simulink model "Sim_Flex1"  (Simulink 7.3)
settings: Solver=ode23  StartTime=0.0  StopTime=120  FixedStep=Ts  RelTol=1e-3
InitFcn:
  | r2d= 180/pi; d2r=1/r2d; Ts=0.04;                  % Radian to degree converts
  | [Afls,Bfls,Cfls,Dfls]= vehicle_flex_s;            % Shuttle Ascent, Max_Q, T=55 sec, Flex Vehicle with Slosh and TWD
  | [Aflz,Bflz,Cflz,Dflz]= vehicle_flex_z;            % Discrete Shuttle Plant Model at Max-Q (Flex Vehicle, Actuators, Sensors)
  | [Alfc,Blfc,Clfc,Dlfc]= lateral_fcs;               % Lateral Flight Control System
  | [Apfc,Bpfc,Cpfc,Dpfc]= pitch_fcs;                 % Pitch Flight Control System
  | [Azpl,Bzpl,Czpl,Dzpl]= vehi_plant_z;              % Load Discrete Plant (Vehi,Actuat,Sensors)
  | [Acts,Bcts,Ccts,Dcts]= actuators_5s;              % System of Five Actuators
  | [Actz,Bctz,Cctz,Dctz]= actuators_5z;              % System of Five Actuators, Z-Transform
  | [Asz, Bsz, Csz, Dsz] = sensors_z;                 % IMU, Gyro, Accelerometer Sensors, Z-transform
  | [Aol, Bol, Col, Dol] = open_loop;                 % Open-Loop System (Plant + FCS)
  | load TVC.Mat -ascii                               % Shuttle Stage-1 TVC Matrix at Max-Q
StopFcn:
  | Pl
undefined symbols (not defined in the file or in its folder): Acts, Afls, Alfc, Apfc, Asz, Bcts, Bfls, Blfc, Bpfc, Bsz, Ccts, Cfls, Clfc, Cpfc, Csz, Dcts, Dfls, Dlfc, Dpfc, Dsz, TVC

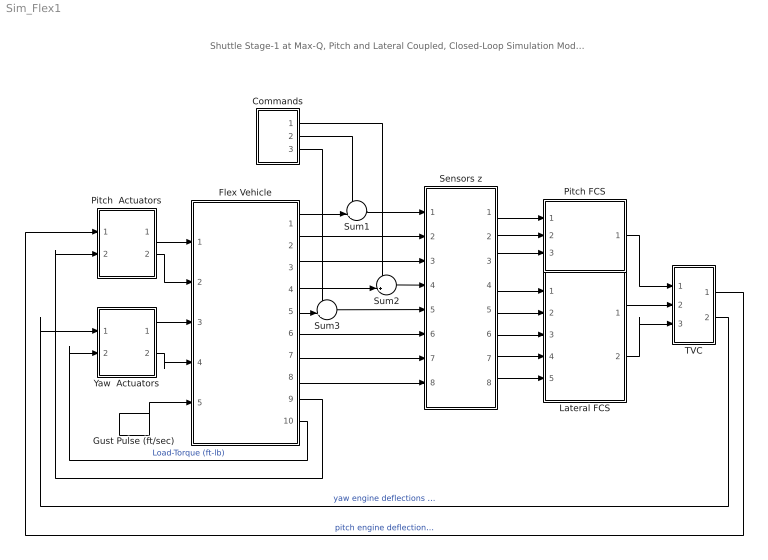
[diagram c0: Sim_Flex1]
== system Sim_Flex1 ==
  note: Shuttle Stage-1 at Max-Q, Pitch and Lateral Coupled, Closed-Loop Simulation Model-1
  Commands : Subsystem
  Flex Vehicle : Subsystem
  Gust Pulse (ft/sec) : DiscretePulseGenerator  PulseType=Time based  Amplitude=30  Period=200  PulseWidth=2.0  PhaseDelay=0.12  SampleTime=1
  Lateral FCS : Subsystem
  Pitch  Actuators : Subsystem
  Pitch FCS : Subsystem
  Sensors z : Subsystem
  Sum1 : Sum  Inputs=-+|  OutDataType=sfix(16)  OutScaling=2^0
  Sum2 : Sum  Inputs=-+|  OutDataType=sfix(16)  OutScaling=2^0
  Sum3 : Sum  Inputs=-+|  OutDataType=sfix(16)  OutScaling=2^0
  TVC : Subsystem
  Yaw  Actuators : Subsystem
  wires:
  Gust Pulse (ft/sec)/1 -> Flex Vehicle/5(WG)
  Flex Vehicle/2(q-flx) -> Sensors z/2(qi)
  Flex Vehicle/3(Nz) -> Sensors z/3(Nzi)
  Flex Vehicle/6(p-flx) -> Sensors z/6(pi)
  Flex Vehicle/7(r-flx) -> Sensors z/7(ri)
  Flex Vehicle/8(Ny) -> Sensors z/8(Nyi)
  Sensors z/1(theo) -> Pitch FCS/1(theta)
  Sensors z/2(qo) -> Pitch FCS/2(q)
  Sensors z/3(Nzo) -> Pitch FCS/3(Nz)
  Sensors z/4(pho) -> Lateral FCS/1(phi-er)
  Sensors z/5(pso) -> Lateral FCS/2(psi-er)
  Sensors z/6(po) -> Lateral FCS/3(p)
  Sensors z/7(ro) -> Lateral FCS/4(r)
  Sensors z/8(Nyo) -> Lateral FCS/5(Ny)
  Pitch  Actuators/1(dy) -> Flex Vehicle/1(dy)
  Yaw  Actuators/1(dz) -> Flex Vehicle/3(dz)
  Yaw  Actuators/2(dzdd) -> Flex Vehicle/4(dzdd)
  Pitch  Actuators/2(dydd) -> Flex Vehicle/2(dydd)
  Flex Vehicle/1(theta) -> Sum1/2
  Sum1/1 -> Sensors z/1(thei)
  Flex Vehicle/4(phi) -> Sum2/2
  Sum2/1 -> Sensors z/4(phi)
  Flex Vehicle/10(TLz) -> Yaw  Actuators/2(TLz)  "Load-Torque (ft-lb)"
  Flex Vehicle/9(TLy) -> Pitch  Actuators/2(TLy)
  Lateral FCS/1(DP_TVC) -> TVC/2(roll)
  Lateral FCS/2(DR_TVC) -> TVC/3(yaw)
  Pitch FCS/1(DQ_TVC) -> TVC/1(ptch)
  TVC/2(dz) -> Yaw  Actuators/1(dzc)  "yaw engine deflections (rad)"
  TVC/1(dy) -> Pitch  Actuators/1(dyc)  "pitch engine deflections (rad)"
  Sum3/1 -> Sensors z/5("psi ")
  Flex Vehicle/5(psi) -> Sum3/2
  Commands/1(roll) -> Sum2/1
  Commands/3(yaw) -> Sum3/1
  Commands/2(ptch) -> Sum1/1

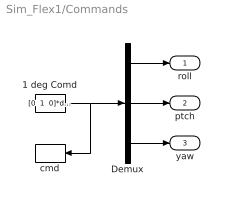
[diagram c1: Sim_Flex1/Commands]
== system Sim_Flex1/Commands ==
  1 deg Comd : Constant  Value="[0  1  0]*d2r"  OutDataType=sfix(16)  OutScaling=2^0  SampleTime=-1
  Demux : Demux  Outputs=3
  cmd : ToWorkspace  VariableName=cmd  SampleTime=-1  SaveFormat=Array
  roll : Outport
  ptch : Outport  Port=2
  yaw : Outport  Port=3
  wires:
  1 deg Comd/1 -> Demux/1, cmd/1
  Demux/1 -> roll/1
  Demux/2 -> ptch/1
  Demux/3 -> yaw/1

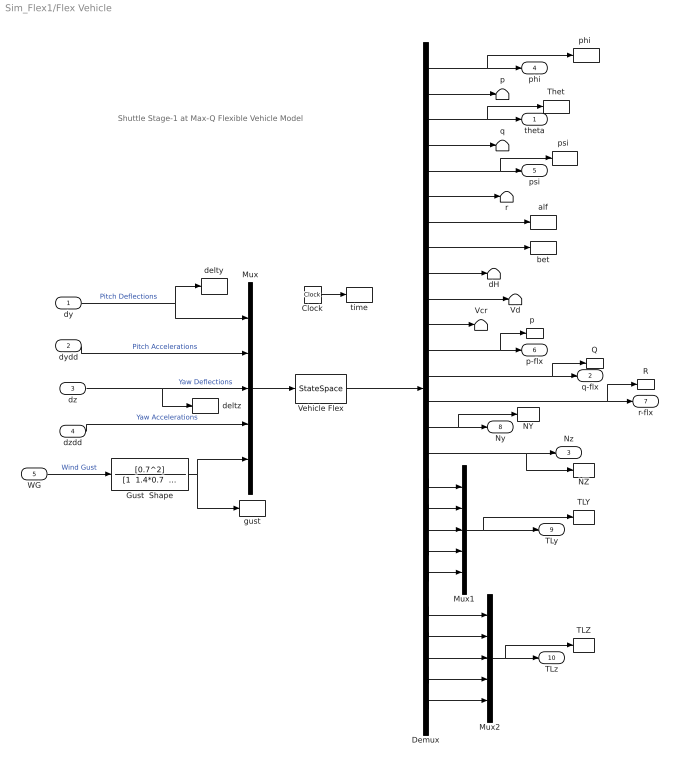
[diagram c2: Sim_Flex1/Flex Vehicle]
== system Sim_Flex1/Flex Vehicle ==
  note: Shuttle Stage-1 at Max-Q Flexible Vehicle Model
  dy : Inport  PortDimensions=5  OutDataType=sfix(16)  OutScaling=2^0
  dydd : Inport  Port=2  PortDimensions=5  OutDataType=sfix(16)  OutScaling=2^0
  dz : Inport  Port=3  PortDimensions=5  OutDataType=sfix(16)  OutScaling=2^0
  dzdd : Inport  Port=4  PortDimensions=5  OutDataType=sfix(16)  OutScaling=2^0
  WG : Inport  Port=5  OutDataType=sfix(16)  OutScaling=2^0
  Clock : Clock
  Demux : Demux  Outputs=26
  Gust  Shape : TransferFcn  Numerator=[0.7^2]  Denominator="[1  1.4*0.7  0.7^2]"
  Mux : Mux  Inputs="[5  5  5  5  1]"
  Mux1 : Mux  Inputs=5
  Mux2 : Mux  Inputs=5
  NY : ToWorkspace  VariableName=Ny  SampleTime=-1  SaveFormat=Array
  NZ : ToWorkspace  VariableName=Nz  SampleTime=-1  SaveFormat=Array
  Q : ToWorkspace  VariableName=q  SampleTime=-1  SaveFormat=Array
  R : ToWorkspace  VariableName=r  SampleTime=-1  SaveFormat=Array
  TLY : ToWorkspace  VariableName=TLy  SampleTime=-1  SaveFormat=Array
  TLZ : ToWorkspace  VariableName=TLz  SampleTime=-1  SaveFormat=Array
  Thet : ToWorkspace  VariableName=theta  SampleTime=-1  SaveFormat=Array
  Vcr : Terminator
  Vd : Terminator
  Vehicle Flex : StateSpace  A=Afls  B=Bfls  C=Cfls  D=Dfls
  alf : ToWorkspace  VariableName=alpha  SampleTime=-1  SaveFormat=Array
  bet : ToWorkspace  VariableName=beta  SampleTime=-1  SaveFormat=Array
  dH : Terminator
  delty : ToWorkspace  VariableName=delty  SampleTime=-1  SaveFormat=Array
  deltz : ToWorkspace  VariableName=deltz  SampleTime=-1  SaveFormat=Array
  gust : ToWorkspace  VariableName=Gust  SampleTime=-1  SaveFormat=Array
  p : Terminator
  "p  " : ToWorkspace  VariableName=p  SampleTime=-1  SaveFormat=Array
  "phi " : ToWorkspace  VariableName=phi  SampleTime=-1  SaveFormat=Array
  "psi " : ToWorkspace  VariableName=psi  SampleTime=-1  SaveFormat=Array
  q : Terminator
  r : Terminator
  time : ToWorkspace  VariableName=time  SampleTime=-1  SaveFormat=Array
  theta : Outport  OutDataType=sfix(16)  OutScaling=2^0
  q-flx : Outport  Port=2  OutDataType=sfix(16)  OutScaling=2^0
  Nz : Outport  Port=3  OutDataType=sfix(16)  OutScaling=2^0
  phi : Outport  Port=4  OutDataType=sfix(16)  OutScaling=2^0
  psi : Outport  Port=5  OutDataType=sfix(16)  OutScaling=2^0
  p-flx : Outport  Port=6  OutDataType=sfix(16)  OutScaling=2^0
  r-flx : Outport  Port=7  OutDataType=sfix(16)  OutScaling=2^0
  Ny : Outport  Port=8  OutDataType=sfix(16)  OutScaling=2^0
  TLy : Outport  Port=9  OutDataType=sfix(16)  OutScaling=2^0
  TLz : Outport  Port=10  OutDataType=sfix(16)  OutScaling=2^0
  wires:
  Mux/1 -> Vehicle Flex/1
  WG/1 -> Gust  Shape/1  "Wind Gust"
  dz/1 -> Mux/3, deltz/1  "Yaw Deflections"
  dydd/1 -> Mux/2  "Pitch Accelerations"
  dy/1 -> Mux/1, delty/1  "Pitch Deflections"
  Demux/1 -> phi/1, "phi "/1
  Demux/5 -> psi/1, "psi "/1
  Demux/2 -> p/1
  Demux/6 -> r/1
  Demux/8 -> bet/1
  Demux/12 -> p-flx/1, "p  "/1
  Demux/13 -> q-flx/1, Q/1
  Demux/15 -> Ny/1, NY/1
  Demux/3 -> theta/1, Thet/1
  Demux/4 -> q/1
  Demux/7 -> alf/1
  Demux/11 -> Vcr/1
  Demux/10 -> Vd/1
  Demux/9 -> dH/1
  Demux/14 -> r-flx/1, R/1
  Demux/16 -> Nz/1, NZ/1
  dzdd/1 -> Mux/4  "Yaw Accelerations"
  Demux/21 -> Mux1/5
  Demux/20 -> Mux1/4
  Demux/19 -> Mux1/3
  Demux/18 -> Mux1/2
  Demux/17 -> Mux1/1
  Demux/22 -> Mux2/1
  Demux/23 -> Mux2/2
  Demux/24 -> Mux2/3
  Demux/25 -> Mux2/4
  Demux/26 -> Mux2/5
  Clock/1 -> time/1
  Mux1/1 -> TLY/1, TLy/1
  Mux2/1 -> TLZ/1, TLz/1
  Gust  Shape/1 -> Mux/5, gust/1
  Vehicle Flex/1 -> Demux/1

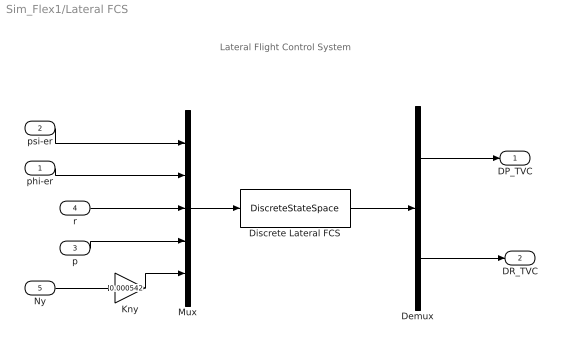
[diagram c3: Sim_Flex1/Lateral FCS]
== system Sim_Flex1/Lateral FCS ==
  note: Lateral Flight Control System
  phi-er : Inport  OutDataType=sfix(16)  OutScaling=2^0
  psi-er : Inport  Port=2  OutDataType=sfix(16)  OutScaling=2^0
  p : Inport  Port=3  OutDataType=sfix(16)  OutScaling=2^0
  r : Inport  Port=4  OutDataType=sfix(16)  OutScaling=2^0
  Ny : Inport  Port=5  OutDataType=sfix(16)  OutScaling=2^0
  Demux : Demux  Outputs=2
  Discrete Lateral FCS : DiscreteStateSpace  A=Alfc  B=Blfc  C=Clfc  D=Dlfc  SampleTime=Ts
  Kny : Gain  Gain=0.000542  ParameterDataType=sfix(16)  ParameterScaling=2^0  OutDataType=sfix(16)  OutScaling=2^0
  Mux : Mux  Inputs=5
  DP_TVC : Outport  OutDataType=sfix(16)  OutScaling=2^0
  DR_TVC : Outport  Port=2  OutDataType=sfix(16)  OutScaling=2^0
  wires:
  psi-er/1 -> Mux/1
  phi-er/1 -> Mux/2
  r/1 -> Mux/3
  Mux/1 -> Discrete Lateral FCS/1
  Discrete Lateral FCS/1 -> Demux/1
  Demux/1 -> DP_TVC/1
  Demux/2 -> DR_TVC/1
  p/1 -> Mux/4
  Ny/1 -> Kny/1
  Kny/1 -> Mux/5

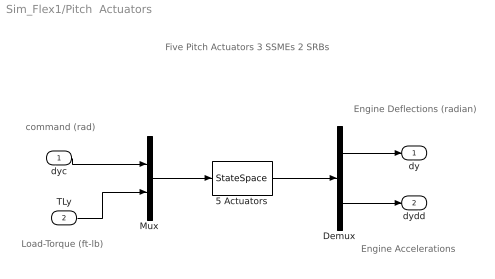
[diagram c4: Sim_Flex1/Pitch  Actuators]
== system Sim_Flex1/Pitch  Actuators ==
  note: Engine Accelerations
  note: Engine Deflections (radian)
  note: Five Pitch Actuators 3 SSMEs 2 SRBs
  note: Load-Torque (ft-lb)
  note: command (rad)
  dyc : Inport  OutDataType=sfix(16)  OutScaling=2^0
  TLy : Inport  Port=2  OutDataType=sfix(16)  OutScaling=2^0
  5 Actuators : StateSpace  A=Acts  B=Bcts  C=Ccts  D=Dcts
  Demux : Demux  Outputs=[5, 5]
  Mux : Mux  Inputs="[5  5]"
  dy : Outport  OutDataType=sfix(16)  OutScaling=2^0
  dydd : Outport  Port=2  OutDataType=sfix(16)  OutScaling=2^0
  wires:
  Mux/1 -> 5 Actuators/1
  dyc/1 -> Mux/1
  TLy/1 -> Mux/2
  Demux/1 -> dy/1
  Demux/2 -> dydd/1
  5 Actuators/1 -> Demux/1

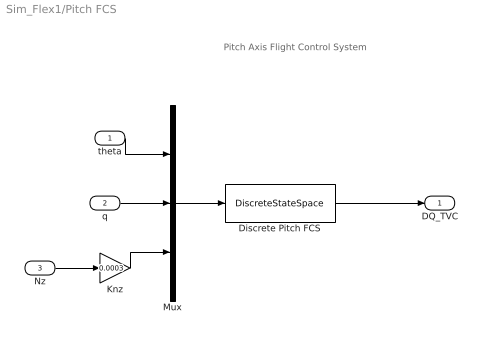
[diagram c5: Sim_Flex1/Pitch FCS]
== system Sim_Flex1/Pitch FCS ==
  note: Pitch Axis Flight Control System
  theta : Inport  OutDataType=sfix(16)  OutScaling=2^0
  q : Inport  Port=2  OutDataType=sfix(16)  OutScaling=2^0
  Nz : Inport  Port=3  OutDataType=sfix(16)  OutScaling=2^0
  Discrete Pitch FCS : DiscreteStateSpace  A=Apfc  B=Bpfc  C=Cpfc  D=Dpfc  SampleTime=Ts
  Knz : Gain  Gain=0.0003  ParameterDataType=sfix(16)  ParameterScaling=2^0  OutDataType=sfix(16)  OutScaling=2^0
  Mux : Mux  Inputs=3
  DQ_TVC : Outport  OutDataType=sfix(16)  OutScaling=2^0
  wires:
  Mux/1 -> Discrete Pitch FCS/1
  Nz/1 -> Knz/1
  q/1 -> Mux/2
  theta/1 -> Mux/1
  Discrete Pitch FCS/1 -> DQ_TVC/1
  Knz/1 -> Mux/3

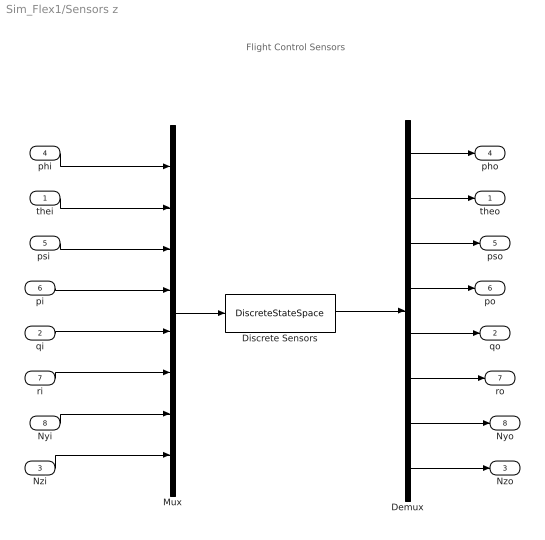
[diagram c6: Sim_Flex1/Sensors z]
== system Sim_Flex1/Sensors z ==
  note: Flight Control Sensors
  thei : Inport  PortDimensions=1  OutDataType=sfix(16)  OutScaling=2^0
  qi : Inport  Port=2  PortDimensions=1  OutDataType=sfix(16)  OutScaling=2^0
  Nzi : Inport  Port=3  PortDimensions=1  OutDataType=sfix(16)  OutScaling=2^0
  phi : Inport  Port=4  PortDimensions=1  OutDataType=sfix(16)  OutScaling=2^0
  "psi " : Inport  Port=5  PortDimensions=1  OutDataType=sfix(16)  OutScaling=2^0
  pi : Inport  Port=6  PortDimensions=1  OutDataType=sfix(16)  OutScaling=2^0
  ri : Inport  Port=7  PortDimensions=1  OutDataType=sfix(16)  OutScaling=2^0
  Nyi : Inport  Port=8  PortDimensions=1  OutDataType=sfix(16)  OutScaling=2^0
  Demux : Demux  Outputs=8
  Discrete Sensors : DiscreteStateSpace  A=Asz  B=Bsz  C=Csz  D=Dsz  SampleTime=Ts
  Mux : Mux  Inputs=8
  theo : Outport  OutDataType=sfix(16)  OutScaling=2^0
  qo : Outport  Port=2  OutDataType=sfix(16)  OutScaling=2^0
  Nzo : Outport  Port=3  OutDataType=sfix(16)  OutScaling=2^0
  pho : Outport  Port=4  OutDataType=sfix(16)  OutScaling=2^0
  pso : Outport  Port=5  OutDataType=sfix(16)  OutScaling=2^0
  po : Outport  Port=6  OutDataType=sfix(16)  OutScaling=2^0
  ro : Outport  Port=7  OutDataType=sfix(16)  OutScaling=2^0
  Nyo : Outport  Port=8  OutDataType=sfix(16)  OutScaling=2^0
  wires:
  Mux/1 -> Discrete Sensors/1
  Discrete Sensors/1 -> Demux/1
  phi/1 -> Mux/1
  thei/1 -> Mux/2
  "psi "/1 -> Mux/3
  pi/1 -> Mux/4
  qi/1 -> Mux/5
  ri/1 -> Mux/6
  Nyi/1 -> Mux/7
  Nzi/1 -> Mux/8
  Demux/1 -> pho/1
  Demux/2 -> theo/1
  Demux/3 -> pso/1
  Demux/4 -> po/1
  Demux/5 -> qo/1
  Demux/6 -> ro/1
  Demux/7 -> Nyo/1
  Demux/8 -> Nzo/1

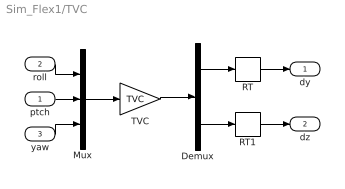
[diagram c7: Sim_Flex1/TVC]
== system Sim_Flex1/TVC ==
  ptch : Inport  OutDataType=sfix(16)  OutScaling=2^0
  roll : Inport  Port=2  OutDataType=sfix(16)  OutScaling=2^0
  yaw : Inport  Port=3  OutDataType=sfix(16)  OutScaling=2^0
  Demux : Demux  Outputs="[5  5]"
  Mux : Mux  Inputs=3
  RT : RateTransition  OutPortSampleTime=Ts
  RT1 : RateTransition  OutPortSampleTime=Ts
  TVC : Gain  Gain=TVC  Multiplication=Matrix(K*u) (u vector)  ParameterDataType=sfix(16)  ParameterScaling=2^0  OutDataType=sfix(16)  OutScaling=2^0
  dy : Outport  OutDataType=sfix(16)  OutScaling=2^0
  dz : Outport  Port=2  OutDataType=sfix(16)  OutScaling=2^0
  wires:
  TVC/1 -> Demux/1
  Mux/1 -> TVC/1
  roll/1 -> Mux/1
  Demux/1 -> RT/1
  ptch/1 -> Mux/2
  Demux/2 -> RT1/1
  yaw/1 -> Mux/3
  RT1/1 -> dz/1
  RT/1 -> dy/1

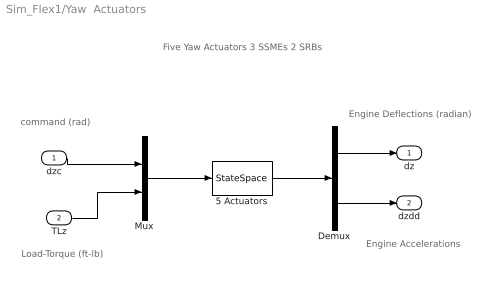
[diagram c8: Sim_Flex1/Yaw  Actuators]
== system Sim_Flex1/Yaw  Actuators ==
  note: Engine Accelerations
  note: Five Yaw Actuators 3 SSMEs 2 SRBs
  note: Engine Deflections (radian)
  note: Load-Torque (ft-lb)
  note: command (rad)
  dzc : Inport  OutDataType=sfix(16)  OutScaling=2^0
  TLz : Inport  Port=2  OutDataType=sfix(16)  OutScaling=2^0
  5 Actuators : StateSpace  A=Acts  B=Bcts  C=Ccts  D=Dcts
  Demux : Demux  Outputs=[5, 5]
  Mux : Mux  Inputs="[5  5]"
  dz : Outport  OutDataType=sfix(16)  OutScaling=2^0
  dzdd : Outport  Port=2  OutDataType=sfix(16)  OutScaling=2^0
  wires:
  Mux/1 -> 5 Actuators/1
  dzc/1 -> Mux/1
  TLz/1 -> Mux/2
  Demux/1 -> dz/1
  Demux/2 -> dzdd/1
  5 Actuators/1 -> Demux/1
